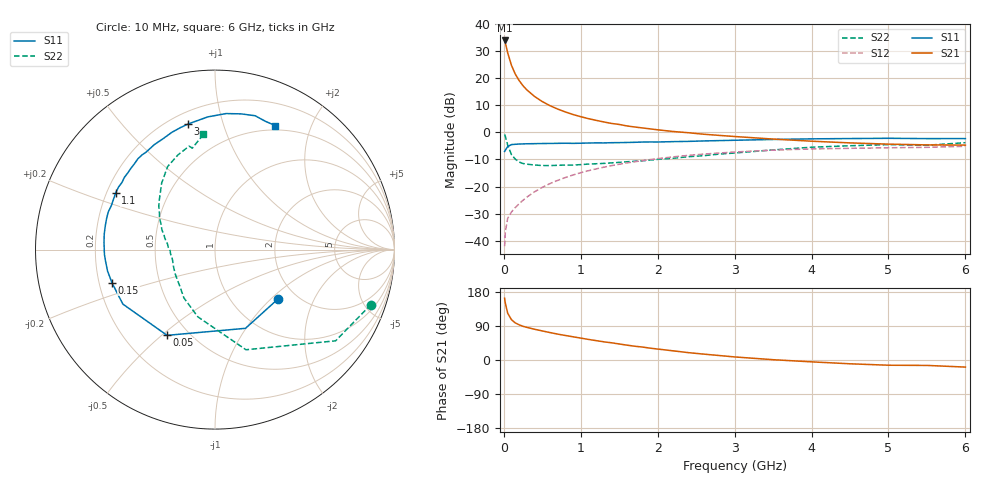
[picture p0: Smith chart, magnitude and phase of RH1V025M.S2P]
! SIEMENS Small Signal Semiconductors
! BFR106
! Si NPN RF Bipolar Junction Transistor in SOT23
! VCE = 1 V  IC = 25 mA
! Common Emitter S-Parameters:  August  1996
# GHz  S  MA  R  50
!  f  S11  S21  S12  S22
! GHz  MAG  ANG  MAG  ANG  MAG  ANG  MAG  ANG
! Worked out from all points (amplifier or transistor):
!   36 points, 10 MHz to 6 GHz, reference 50 ohm
!   highest |S21| = 34.0 dB at 10 MHz (marker M1)
!   |S21| within 3 dB of that: start of sweep to 37.12 MHz
!   unconditionally stable (mu >= 1): 297.8 MHz to 3.45 GHz; 3.698 GHz to end of sweep
!   at 250 MHz: K = 0.96, MSG = 21.1 dB, |S12| = -25.1 dB
!   at 1.4 GHz: K = 1.08, MAG = 6.0 dB, |S12| = -12.3 dB
!   at 6 GHz: K = 1.02, MAG = -0.7 dB, |S12| = -5.1 dB
!   S11 on the Smith chart (normalised r, x): 10 MHz: 1.60, -1.11; 50 MHz: 0.38, -0.52; 150 MHz: 0.25, -0.15; 1.1 GHz: 0.24, +0.25; 3 GHz: 0.27, +0.77; 6 GHz: 0.45, +1.50
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0.01  0.4455 -38.4  50.03 163.0  0.0079 78.1  0.9214 -19.4
0.02  0.4704 -68.8  44.98 149.3  0.0147 67.6  0.8425 -37.1
0.05  0.5473 -119.2  29.59 123.5  0.0259 51.9  0.5842 -72.8
0.1  0.5964 -149.4  17.22 106.1  0.034 49.3  0.3866 -104.3
0.15  0.6032 -162.2  11.86 97.8  0.041 51.9  0.32 -122.8
0.2  0.6104 -168.7  9.042 92.8  0.0483 55.6  0.2826 -134.0
0.25  0.6132 -174.0  7.246 88.9  0.0558 58.0  0.2663 -143.3
0.3  0.6166 -177.5  6.078 86.1  0.0639 60.6  0.2591 -149.1
0.4  0.6195 176.5  4.612 81.1  0.08 62.9  0.2494 -158.3
0.5  0.6232 172.1  3.711 76.7  0.0965 64.0  0.2445 -164.3
0.6  0.6253 167.9  3.118 72.4  0.1133 64.0  0.2436 -168.2
0.7  0.6281 164.1  2.701 68.3  0.1299 63.7  0.2467 -171.8
0.9  0.6273 157.1  2.14 61.2  0.1635 61.9  0.2495 -178.3
1.1  0.6368 150.4  1.795 54.3  0.1959 59.4  0.2598 177.6
1.3  0.6392 144.2  1.559 48.0  0.2277 56.4  0.2675 172.9
1.6  0.652 135.7  1.318 39.2  0.2729 51.6  0.2868 167.0
2.2  0.6755 120.1  1.04 24.2  0.3531 41.6  0.3324 154.7
3  0.7158 102.1  0.84 8.1  0.4341 28.0  0.4161 138.2
3.5  0.7405 93.1  0.753 0.8  0.4708 20.3  0.4747 128.8
4.5  0.7701 79.1  0.64 -10.0  0.5083 6.3  0.5668 111.3
5.5  0.7679 68.5  0.588 -14.3  0.5298 -1.9  0.579 102.6
6  0.7683 64.1  0.582 -18.7  0.5529 -8.6  0.6461 95.7
